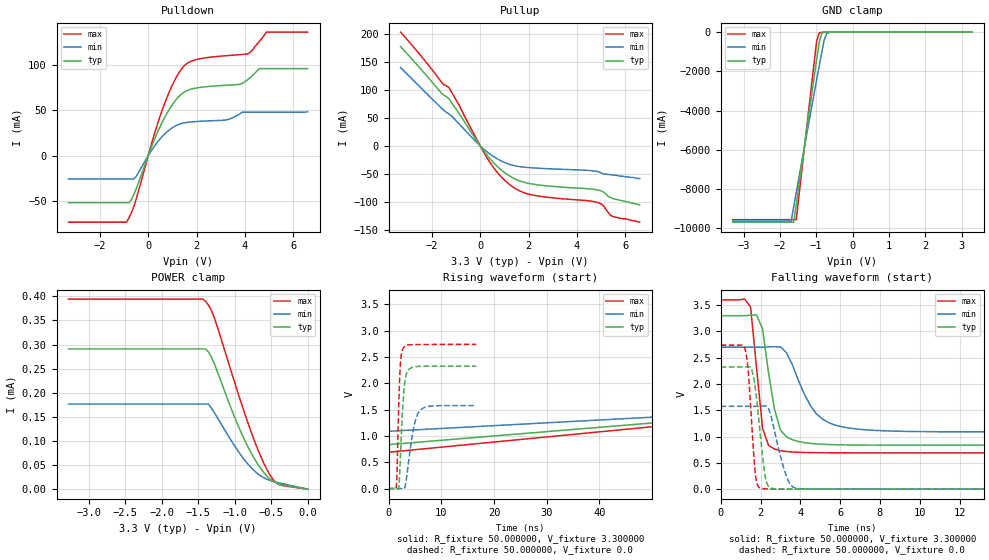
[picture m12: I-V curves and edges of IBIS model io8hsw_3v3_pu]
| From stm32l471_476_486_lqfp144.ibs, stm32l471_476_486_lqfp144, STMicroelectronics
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|   Model io8hsw_3v3_pu
[Model]  io8hsw_3v3_pu
Model_type I/O
Polarity   Non-Inverting
Enable   Active-Low
Vinl =   0.990000V
Vinh =   2.310000V
Vmeas =  1.650000V
Cref =   100.000000nF
Rref =   1.000000k
Vref =   3.300000V
C_comp   2.968600pF   2.938100pF   3.196200pF
[Temperature Range]   25.000000   0.125000k   -40.000000
[Pullup Reference]   3.300000V   2.700000V   3.600000V
[Pulldown Reference]   0.0V   0.0V   0.0V
[POWER Clamp Reference]   3.300000V   2.700000V   3.600000V
[GND Clamp Reference]   0.0V   0.0V   0.0V
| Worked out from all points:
|   slope of the pulldown table from 0 to 0.495 V, typ, clamps not added: 15.4 ohm
|   slope of the pullup table from 0 to 0.495 V, typ, clamps not added: 18.1 ohm
|   GND clamp passes 1 mA (typ) near -0.58 V on its own axis
|   rising waveform, R_fixture 50.000000, V_fixture 3.300000: 20-80 % time 180ns typ, 180ns min, 180ns max; typ from 0.836 V to 3.3 V
|   rising waveform, R_fixture 50.000000, V_fixture 0.0: 20-80 % time 725ps typ, 1.46ns min, 488ps max; typ from 0.001 V to 2.33 V
|   falling waveform, R_fixture 50.000000, V_fixture 3.300000: 20-80 % time 659ps typ, 1.29ns min, 455ps max; typ from 3.3 V to 0.836 V
|   falling waveform, R_fixture 50.000000, V_fixture 0.0: 20-80 % time 392ps typ, 627ps min, 287ps max; typ from 2.33 V to 0.001 V
[Pulldown]
|Voltage   I(typ)   I(min)   I(max)
-3.3V     -51.62mA   -25.53mA   -73.04mA
-900mV    -51.62mA   -25.53mA   -73.04mA
-500mV    -36.51mA   -22.79mA   -47.71mA
200mV     14.02mA    8.316mA    18.9mA
700mV     42.98mA    24.4mA     58.9mA
1.2V      63.06mA    33.8mA     88.14mA
1.6V      71.63mA    36.67mA    101.4mA
3.2V      77.51mA    39.29mA    110mA
4.1V      83.28mA    47.99mA    112mA
4.6V      95.81mA    47.99mA    125.7mA
4.9V      95.81mA    47.99mA    136mA
6.6V      95.81mA    48.43mA    136mA
[Pullup]
|Voltage   I(typ)   I(min)   I(max)
-3.3V     177.3mA    140mA      203.2mA
-1.6V     93.97mA    67.34mA    113.5mA
-1.3V     83.99mA    57.44mA    104.3mA
300mV     -17.49mA   -11.19mA   -22.71mA
700mV     -36.32mA   -22.9mA    -46.84mA
1.2V      -53.2mA    -32.62mA   -68.33mA
1.7V      -63.36mA   -37.26mA   -81.47mA
2.2V      -68.23mA   -39.11mA   -87.81mA
4.8V      -78.1mA    -45mA      -100.2mA
5.1V      -82mA      -50mA      -106.7mA
5.5V      -94mA      -52mA      -126mA
6.6V      -105mA     -58mA      -136mA
[GND_clamp]
|Voltage   I(typ)   I(min)   I(max)
-3.3V     -9.687A    -9.633A    -9.557A
-1.69V    -9.687A    -9.633A    -9.557A
-1.62V    -9.687A    -8.894A    -9.557A
-1.55V    -8.764A    -8.167A    -9.557A
-1.13V    -3.236A    -3.867A    -2.713A
-990mV    -1.416A    -2.448A    -480.1mA
-920mV    -530mA     -1.746A    -39.96mA
-850mV    -62.36mA   -1.055A    -14.04mA
-780mV    -12.04mA   -390.4mA   -9.013mA
-710mV    -4.897mA   -69.08mA   -5.32mA
-640mV    -2.305mA   -14.59mA   -2.498mA
3.28V     0A         0A         0A
[POWER_clamp]
|Voltage   I(typ)   I(min)   I(max)
-3.28V    291uA      176.5uA    394.3uA
-1.44V    291uA      176.5uA    394.3uA
-1.4V     291uA      176.5uA    389.8uA
-1.36V    284.6uA    176.5uA    382.1uA
-1.28V    260.2uA    158.7uA    355.4uA
-1V       148.8uA    89.45uA    220.9uA
-840mV    94.39uA    55.87uA    146.9uA
-680mV    51.08uA    31.49uA    81.3uA
-560mV    27.28uA    20.64uA    41.26uA
-480mV    16.8uA     16.48uA    21.17uA
-400mV    11.23uA    13.43uA    10.02uA
0V        0A         5.022nA    0A
[Ramp]
| variable   typ   min   max
dV/dt_r  1.39438/0.72441n   0.94482/1.45633n   1.64276/0.48777n
dV/dt_f  1.47812/0.60362n   0.96630/1.27330n   1.74547/0.39887n
R_load = 50.000000
[Rising Waveform]
R_fixture= 50.000000
V_fixture= 3.300000
V_fixture_min= 2.700000
V_fixture_max= 3.600000
|time   V(typ)   V(min)   V(max)
0s        836mV      1.089V     690.6mV
300.3ns   3.3V       2.7V       3.6V
600.6ns   3.3V       2.7V       3.6V
29.73us   3.3V       2.7V       3.6V
[Rising Waveform]
R_fixture= 50.000000
V_fixture= 0.0
V_fixture_min= 0.0
V_fixture_max= 0.0
|time   V(typ)   V(min)   V(max)
0s        932.4uV    1.4mV      660.9uV
1.468ns   1.222mV    1.4mV      41.33mV
1.568ns   -169.6uV   1.4mV      206.7mV
1.935ns   31.61mV    1.427mV    1.629V
2.169ns   433.1mV    1.513mV    2.249V
2.769ns   1.671V     -8.152mV   2.663V
3.504ns   2.209V     283.3mV    2.722V
4.705ns   2.31V      1.127V     2.736V
5.873ns   2.322V     1.472V     2.738V
16.62ns   2.325V     1.576V     2.739V
[Falling Waveform]
R_fixture= 50.000000
V_fixture= 3.300000
V_fixture_min= 2.700000
V_fixture_max= 3.600000
|time   V(typ)   V(min)   V(max)
0s        3.3V       2.7V       3.6V
1.502ns   3.309V     2.7V       3.465V
1.802ns   3.314V     2.7V       2.305V
2.102ns   3.05V      2.7V       1.159V
2.402ns   2.214V     2.709V     833.9mV
3.003ns   1.125V     2.706V     732.7mV
3.604ns   939.7mV    2.363V     707.9mV
5.105ns   854.8mV    1.337V     693.6mV
9.009ns   837.2mV    1.102V     691.3mV
149.5ns   836mV      1.089V     690.6mV
[Falling Waveform]
R_fixture= 50.000000
V_fixture= 0.0
V_fixture_min= 0.0
V_fixture_max= 0.0
|time   V(typ)   V(min)   V(max)
0s        2.325V     1.576V     2.739V
1.235ns   2.325V     1.576V     2.65V
1.401ns   2.331V     1.576V     2.16V
1.735ns   1.939V     1.576V     311.6mV
1.969ns   1.114V     1.577V     22.74mV
2.202ns   324.8mV    1.584V     7.337mV
2.369ns   73.17mV    1.552V     4.676mV
3.27ns    4.474mV    280.8mV    2.241mV
3.737ns   2.983mV    23.33mV    1.836mV
16.62ns   932.4uV    1.4mV      660.9uV
